| IBIS file stm32mp211_213_215_vfbga225.ibs
[IBIS ver] 5.1
[File name] stm32mp211_213_215_vfbga225.ibs
[File Rev] 0.4
[Date] 09-10-2025
[Source] Data Created at STMicroelectronics
[Notes]  File originated from ELDO simulations.
[Disclaimer]  This information is for modeling purpose only and is
   not guaranted. The information is subject to change without
   notice.
[Copyright] Copyright 2025 STMicroelectronics Inc.
|   Component stm32mp211_213_215_vfbga225
[Component] stm32mp211_213_215_vfbga225
[Manufacturer] STMicroelectronics
[Package]
| variable   typ   min   max
R_pkg  0  NA  NA
L_pkg  0  NA  NA
C_pkg  0  NA  NA
[Pin]   signal_name   model_name
A1  VSS  gnd
A2  PG5  io8_tt
A3  PG11  io8_tt
A4  PD3  io8_tt
A5  PD4  io8_tt
A6  PD15  io8_tt_i3c
A7  PE5  io8_tt
A8  PE3  io8_tt
A9  PE8  io8_tt
A10  PE13  io8_tt
A11  PE12  io8_tt
A12  PB14  io8_tt
A13  PD12  io8_tt
A14  PD13  io8_tt
A15  VSS  gnd
B1  PG7  io8_tt
B2  PI1  io8_tt_i3c
B3  PF15  io8_tt
B4  PD10  io8_tt_i3c
B5  PB11  io8_tt
B6  PD8  io8_tt
B7  PE1  io8_tt
B8  PE4  io8_tt
B9  PE15  io8_tt
B10  PE7  io8_tt
B11  PE9  io8_tt
B12  PB13  io8_tt
B13  PB12  io8_tt
B14  DDR_A20  mal4drv20_PAD
B15  DDR_DQ11  mal4drv27_PAD
C1  PF12  io8_tt
C2  PI4  io8_tt
C3  PF13  io8_tt
C4  PD2  io8_tt
C5  PD11  io8_tt_i3c
C6  PD1  io8_tt
C7  PD9  io8_tt
C8  PE0  io8_tt
C9  PE2  io8_tt
C10  PE11  io8_tt
C11  PD14  io8_tt
C12  DDR_RESETN  nc
C13  DDR_A9  mal4drv20_PAD
C14  DDR_A21  mal4drv20_PAD
C15  DDR_DQ9  mal4drv27_PAD
D1  OSC_OUT  isudq_v18
D2  OSC_IN  isudq_v18
D3  PI0  io8_tt
D4  PG12  io8_tt
D5  PD0  io8_tt
D6  PD7  io8_tt
D7  PD5  io8_tt
D8  PD6  io8_tt
D9  VDDA18PLL1  nc
D10  PE6  io8_tt
D11  DDR_A3  mal4drv20_PAD
D12  DDR_DQ10  mal4drv27_PAD
D13  DDR_A11  mal4drv20_PAD
D14  DDR_A22  mal4drv20_PAD
D15  DDR_DQS1N  mal4drv27_PAD
E1  OSC32_IN  isudq_v18
E2  OSC32_OUT  isudq_v18
E3  BOOT0  isudq_tt
E4  PC13  io8_tt
E5  VDDA18PLL2  nc
E6  VDDIO3  power
E7  VDDIO3  power
E8  VDDIO2  power
E9  VDDIO1  power
E10  VDDA18DDR  nc
E11  DDR_A0  mal4drv20_PAD
E12  DDR_DQ8  mal4drv27_PAD
E13  DDR_A10  mal4drv20_PAD
E14  DDR_A23  mal4drv20_PAD
E15  DDR_DQS1P  mal4drv27_PAD
F1  BOOT1  isudq_tt
F2  NRSTC1MS  io8_tt
F3  PWR_ON  io8_tt
F4  VDDA18AON  power
F5  VSSAON  nc
F6  VSS  gnd
F7  VDDCPU  nc
F8  VSS  gnd
F9  VDDCPU  nc
F10  VSS  gnd
F11  DDR_A5  mal4drv20_PAD
F12  DDR_A1  mal4drv20_PAD
F13  DDR_A8  mal4drv20_PAD
F14  DDR_A25  mal4drv20_PAD
F15  DDR_DQM1  mal4drv27_PAD
G1  JTDO_TRACESWO  io8_tt
G2  BOOT3  isudq_tt
G3  BOOT2  isudq_tt
G4  PDR_ON  nc
G5  V08CAP  nc
G6  VDDCORE  nc
G7  VSS  gnd
G8  VDDCPU  nc
G9  VSS  gnd
G10  VDDQDDR  power
G11  DDR_A4  mal4drv20_PAD
G12  DDR_DQ15  mal4drv27_PAD
G13  DDR_A14  mal4drv20_PAD
G14  DDR_A26  mal4drv20_PAD
G15  DDR_DQ12  mal4drv27_PAD
H1  JTCK_SWCLK  io8_tt
H2  NRST  nc
H3  PWR_LP  io8_tt
H4  PWR_CPUON  io8_tt
H5  VBAT  power
H6  VSS  gnd
H7  VDDCORE  nc
H8  VSS  gnd
H9  VDDQDDR  power
H10  VSS  gnd
H11  DDR_VREF  nc
H12  DDR_DQ5  mal4drv27_PAD
H13  DDR_DQ14  mal4drv27_PAD
H14  DDR_DQ13  mal4drv27_PAD
H15  DDR_DQ4  mal4drv27_PAD
J1  JTMS_SWDIO  io8_tt
J2  NJTRST  io8_tt
J3  JTDI  io8_tt
J4  VDDA18ADC  power
J5  VSSA  nc
J6  VDD  power
J7  VSS  gnd
J8  VDDCORE  nc
J9  VSS  gnd
J10  VDDQDDR  power
J11  DDR_A6  mal4drv20_PAD
J12  VSS  gnd
J13  DDR_ZQ  nc
J14  DDR_A13  mal4drv20_PAD
J15  DDR_DQ6  mal4drv27_PAD
K1  VREFN  nc
K2  PG2  io8_tt_i3c
K3  PA0  io8_tt
K4  PG3  io8_tt
K5  VDD  power
K6  VSS  gnd
K7  VDD  power
K8  VSS  gnd
K9  VDDCORE  nc
K10  VSS  gnd
K11  DDR_A18  mal4drv20_PAD
K12  DDR_DQ7  mal4drv27_PAD
K13  DDR_A27  mal4drv20_PAD
K14  DDR_A2  mal4drv20_PAD
K15  DDR_DQS0P  mal4drv27_PAD
L1  VREFP  nc
L2  PF11  io8_tt
L3  PG4  io8_tt
L4  PC8  io8_tt
L5  PF3  io8_tt
L6  PC0  io8_tt
L7  PH13  io8_tt
L8  PH11  io8_tt
L9  PA9  io8_tt
L10  VDDQDDR  power
L11  DDR_A31  mal4drv20_PAD
L12  DDR_A7  mal4drv20_PAD
L13  DDR_A28  mal4drv20_PAD
L14  DDR_A15  mal4drv20_PAD
L15  DDR_DQS0N  mal4drv27_PAD
M1  PB15  io8_tt
M2  PG1  io8_tt_i3c
M3  PC3  io8_tt
M4  PC9  io8_tt
M5  PC4  io8_tt
M6  PA15  io8_tt_i3c
M7  PA14  io8_tt
M8  PF0  io8_tt_i3c
M9  PA5  io8_tt
M10  PA2  io8_tt_i3c
M11  DDR_A12  mal4drv20_PAD
M12  DDR_DQM0  mal4drv27_PAD
M13  DDR_A29  mal4drv20_PAD
M14  DDR_A16  mal4drv20_PAD
M15  DDR_DQ0  mal4drv27_PAD
N1  PF4  io8_tt
N2  PF6  io8_tt
N3  PA10  io8_tt
N4  PF5  io8_tt
N5  PF8  io8_tt
N6  PC2  io8_tt
N7  PH9  io8_tt
N8  PA13  io8_tt
N9  PA8  io8_tt_i3c
N10  PA1  io8_tt_i3c
N11  DDR_DQ3  mal4drv27_PAD
N12  DDR_DQ2  mal4drv27_PAD
N13  DDR_A30  mal4drv20_PAD
N14  DDR_A17  mal4drv20_PAD
N15  DDR_DQ1  mal4drv27_PAD
P1  PF9  io8_tt
P2  PH4  io8_tt
P3  PF10  io8_tt
P4  PG0  io8_tt_i3c
P5  PF7  io8_tt
P6  PC5  io8_tt_i3c
P7  PC6  io8_tt_i3c
P8  PF2  io8_tt_i3c
P9  PH12  io8_tt
P10  PA7  io8_tt
P11  PH5  io8_tt
P12  PA3  io8_tt_i3c
P13  VSS  gnd
P14  OTG_HSDP  USB2_HS_IBIS
P15  VDD33USB  power
R1  VSS  gnd
R2  PC12  io8_tt_i3c
R3  PC11  io8_tt
R4  PA11  io8_tt
R5  PC7  io8_tt
R6  PC10  io8_tt
R7  PC1  io8_tt_i3c
R8  PF1  io8_tt
R9  PH10  io8_tt
R10  PA6  io8_tt
R11  PA4  io8_tt
R12  VDDA18USB  nc
R13  OTG_TXRTUNE  nc
R14  OTG_HSDM  USB2_HS_IBIS
R15  VSS  gnd
[Package Model]   503-fcvfbga-8x8-225-240814
[Pin Mapping]   pulldown_ref   pullup_ref   | Comment
A1  gnd  nc
A2  gnd  vdd
A3  gnd  vdd
A4  gnd  vddio3
A5  gnd  vddio3
A6  gnd  vdd
A7  gnd  vddio1
A8  gnd  vddio1
A9  gnd  vddio1
A10  gnd  vddio2
A11  gnd  vddio2
A12  gnd  vdd
A13  gnd  vdd
A14  gnd  vdd
A15  gnd  nc
B1  gnd  vdd
B2  gnd  vdd
B3  gnd  vdd
B4  gnd  vddio3
B5  gnd  vdd
B6  gnd  vddio3
B7  gnd  vddio1
B8  gnd  vddio1
B9  gnd  vddio2
B10  gnd  vddio1
B11  gnd  vddio1
B12  gnd  vdd
B13  gnd  vdd
B14  gnd  vddqddr
B15  gnd  vddqddr
C1  gnd  vdd
C2  gnd  vdd
C3  gnd  vdd
C4  gnd  vddio3
C5  gnd  vddio3
C6  gnd  vddio3
C7  gnd  vddio3
C8  gnd  vddio1
C9  gnd  vddio1
C10  gnd  vddio2
C11  gnd  vdd
C12  nc  nc
C13  gnd  vddqddr
C14  gnd  vddqddr
C15  gnd  vddqddr
D1  gnd  vdda18aon
D2  gnd  vdda18aon
D3  gnd  vdd
D4  gnd  vdd
D5  gnd  vddio3
D6  gnd  vddio3
D7  gnd  vddio3
D8  gnd  vddio3
D9  nc  nc
D10  gnd  vddio1
D11  gnd  vddqddr
D12  gnd  vddqddr
D13  gnd  vddqddr
D14  gnd  vddqddr
D15  gnd  vddqddr
E1  gnd  vdd  | Depending on IO usage
| E1  gnd  vsw  | Depending on IO usage
E2  gnd  vdd  | Depending on IO usage
| E2  gnd  vsw  | Depending on IO usage
E3  gnd  vdd
E4  gnd  vdd  | Depending on IO usage
| E4  gnd  vsw  | Depending on IO usage
E5  nc  nc
E6  nc  vddio3
E7  nc  vddio3
E8  nc  vddio2
E9  nc  vddio1
E10  nc  nc
E11  gnd  vddqddr
E12  gnd  vddqddr
E13  gnd  vddqddr
E14  gnd  vddqddr
E15  gnd  vddqddr
F1  gnd  vdd
F2  gnd  vdd
F3  gnd  vdd
F4  nc  vdda18aon
F5  nc  nc
F6  gnd  nc
F7  nc  nc
F8  gnd  nc
F9  nc  nc
F10  gnd  nc
F11  gnd  vddqddr
F12  gnd  vddqddr
F13  gnd  vddqddr
F14  gnd  vddqddr
F15  gnd  vddqddr
G1  gnd  vdd
G2  gnd  vdd
G3  gnd  vdd
G4  nc  nc
G5  nc  nc
G6  nc  nc
G7  gnd  nc
G8  nc  nc
G9  gnd  nc
G10  nc  vddqddr
G11  gnd  vddqddr
G12  gnd  vddqddr
G13  gnd  vddqddr
G14  gnd  vddqddr
G15  gnd  vddqddr
H1  gnd  vdd
H2  nc  nc
H3  gnd  vdd
H4  gnd  vdd
H5  nc  vsw
H6  gnd  nc
H7  nc  nc
H8  gnd  nc
H9  nc  vddqddr
H10  gnd  nc
H11  nc  nc
H12  gnd  vddqddr
H13  gnd  vddqddr
H14  gnd  vddqddr
H15  gnd  vddqddr
J1  gnd  vdd
J2  gnd  vdd
J3  gnd  vdd
J4  nc  vdda18adc
J5  nc  nc
J6  nc  vdd
J7  gnd  nc
J8  nc  nc
J9  gnd  nc
J10  nc  vddqddr
J11  gnd  vddqddr
J12  gnd  nc
J13  nc  nc
J14  gnd  vddqddr
J15  gnd  vddqddr
K1  nc  nc
K2  gnd  vdd
K3  gnd  vdd
K4  gnd  vdd
K5  nc  vdd
K6  gnd  nc
K7  nc  vdd
K8  gnd  nc
K9  nc  nc
K10  gnd  nc
K11  gnd  vddqddr
K12  gnd  vddqddr
K13  gnd  vddqddr
K14  gnd  vddqddr
K15  gnd  vddqddr
L1  nc  nc
L2  gnd  vdd
L3  gnd  vdd
L4  gnd  vdd
L5  gnd  vdd
L6  gnd  vdd
L7  gnd  vdd
L8  gnd  vdd
L9  gnd  vdd
L10  nc  vddqddr
L11  gnd  vddqddr
L12  gnd  vddqddr
L13  gnd  vddqddr
L14  gnd  vddqddr
L15  gnd  vddqddr
M1  gnd  vdd
M2  gnd  vdd
M3  gnd  vdd
M4  gnd  vdd
M5  gnd  vdd
M6  gnd  vdd
M7  gnd  vdd
M8  gnd  vdd
M9  gnd  vdd
M10  gnd  vdd
M11  gnd  vddqddr
M12  gnd  vddqddr
M13  gnd  vddqddr
M14  gnd  vddqddr
M15  gnd  vddqddr
N1  gnd  vdd
N2  gnd  vdd
N3  gnd  vdd
N4  gnd  vdd
N5  gnd  vdd
N6  gnd  vdd
N7  gnd  vdd
N8  gnd  vdd
N9  gnd  vdd
N10  gnd  vdd
N11  gnd  vddqddr
N12  gnd  vddqddr
N13  gnd  vddqddr
N14  gnd  vddqddr
N15  gnd  vddqddr
P1  gnd  vdd
P2  gnd  vdd
P3  gnd  vdd
P4  gnd  vdd
P5  gnd  vdd
P6  gnd  vdd
P7  gnd  vdd
P8  gnd  vdd
P9  gnd  vdd
P10  gnd  vdd
P11  gnd  vdd
P12  gnd  vdd
P13  gnd  nc
P14  gnd  vdd33usb
P15  nc  vdd33usb
R1  gnd  nc
R2  gnd  vdd
R3  gnd  vdd
R4  gnd  vdd
R5  gnd  vdd
R6  gnd  vdd
R7  gnd  vdd
R8  gnd  vdd
R9  gnd  vdd
R10  gnd  vdd
R11  gnd  vdd
R12  nc  nc
R13  nc  nc
R14  gnd  vdd33usb
R15  gnd  nc
[Diff Pin]  inv_pin  vdiff  tdelay_typ  tdelay_min  tdelay_max
K15  L15  NA  NA  NA  NA
E15  D15  NA  NA  NA  NA
G11  F11  NA  NA  NA  NA
P14  R14  NA  NA  NA  NA   |USBH_HS_DP _DM
[Model Selector] USB2_HS_IBIS
USB2_HSRX   USB2 HSRX model
USB2_HSTX_00_0_01_0011_11   TuningBits_AMP_PULSE_RISE_REF_XV=00_0_01_0011_11
USB2_HSTX_00_0_10_0101_11   TuningBits_AMP_PULSE_RISE_REF_XV=00_0_10_0101_11
USB2_HSTX_00_0_11_0111_11   TuningBits_AMP_PULSE_RISE_REF_XV=00_0_11_0111_11
USB2_HSTX_00_1_01_0011_11   TuningBits_AMP_PULSE_RISE_REF_XV=00_1_01_0011_11
USB2_HSTX_00_1_10_0101_11   TuningBits_AMP_PULSE_RISE_REF_XV=00_1_10_0101_11
USB2_HSTX_00_1_11_0111_11   TuningBits_AMP_PULSE_RISE_REF_XV=00_1_11_0111_11
USB2_HSTX_01_0_01_0011_11   TuningBits_AMP_PULSE_RISE_REF_XV=01_0_01_0011_11
USB2_HSTX_01_0_10_0101_11   TuningBits_AMP_PULSE_RISE_REF_XV=01_0_10_0101_11
USB2_HSTX_01_0_11_0111_11   TuningBits_AMP_PULSE_RISE_REF_XV=01_0_11_0111_11
USB2_HSTX_01_1_01_0011_11   TuningBits_AMP_PULSE_RISE_REF_XV=01_1_01_0011_11
USB2_HSTX_01_1_10_0101_11   TuningBits_AMP_PULSE_RISE_REF_XV=01_1_10_0101_11
USB2_HSTX_01_1_11_0111_11   TuningBits_AMP_PULSE_RISE_REF_XV=01_1_11_0111_11
USB2_HSTX_10_0_01_0011_11   TuningBits_AMP_PULSE_RISE_REF_XV=10_0_01_0011_11
USB2_HSTX_10_0_10_0101_11   TuningBits_AMP_PULSE_RISE_REF_XV=10_0_10_0101_11
USB2_HSTX_10_0_11_0111_11   TuningBits_AMP_PULSE_RISE_REF_XV=10_0_11_0111_11
USB2_HSTX_10_1_01_0011_11   TuningBits_AMP_PULSE_RISE_REF_XV=10_1_01_0011_11
USB2_HSTX_10_1_10_0101_11   TuningBits_AMP_PULSE_RISE_REF_XV=10_1_10_0101_11
USB2_HSTX_10_1_11_0111_11   TuningBits_AMP_PULSE_RISE_REF_XV=10_1_11_0111_11
[Model Selector] io8_tt
io8_tt_ls_3v3 "GPIO - 3V tolerant - low speed - 3.3V range"
io8_tt_ms_3v3 "GPIO - 3V tolerant - med speed - 3.3V range"
io8_tt_fs_3v3 "GPIO - 3V tolerant - fast speed - 3.3V range"
io8_tt_hs_3v3 "GPIO - 3V tolerant - high speed - 3.3V range"
io8_tt_hslv_ls_1v8 "GPIO low voltage optimization - 3V tolerant - low speed - 1.8V range"
io8_tt_hslv_ms_1v8 "GPIO low voltage optimization - 3V tolerant - med speed - 1.8V range"
io8_tt_hslv_fs_1v8 "GPIO low voltage optimization - 3V tolerant - fast speed - 1.8V range"
io8_tt_hslv_hs_1v8 "GPIO low voltage optimization - 3V tolerant - high speed - 1.8V range"
[Model Selector] io8_tt_i3c
io8_tt_ls_3v3 "GPIO - 3V tolerant - low speed - 3.3V range"
io8_tt_ms_3v3 "GPIO - 3V tolerant - med speed - 3.3V range"
io8_tt_fs_3v3 "GPIO - 3V tolerant - fast speed - 3.3V range"
io8_tt_hs_3v3 "GPIO - 3V tolerant - high speed - 3.3V range"
io8_tt_hslv_ls_1v8 "GPIO low voltage optimization - 3V tolerant - low speed - 1.8V range"
io8_tt_hslv_ms_1v8 "GPIO low voltage optimization - 3V tolerant - med speed - 1.8V range"
io8_tt_hslv_fs_1v8 "GPIO low voltage optimization - 3V tolerant - fast speed - 1.8V range"
io8_tt_hslv_hs_1v8 "GPIO low voltage optimization - 3V tolerant - high speed - 1.8V range"
io8_tt_i3c_ls_3v3 "GPIO with I3C open-drain - 3V tolerant - low speed - 3.3V range"
io8_tt_i3c_ms_3v3 "GPIO with I3C open-drain - 3V tolerant - med speed - 3.3V range"
io8_tt_i3c_fs_3v3 "GPIO with I3C open-drain - 3V tolerant - fast speed - 3.3V range"
io8_tt_i3c_hs_3v3 "GPIO with I3C open-drain - 3V tolerant - high speed - 3.3V range"
io8_tt_hslv_i3c_ls_1v8 "GPIO low voltage optimization with I3C open-drain - 3V tolerant - low speed - 1.8V range"
io8_tt_hslv_i3c_ms_1v8 "GPIO low voltage optimization with I3C open-drain - 3V tolerant - med speed - 1.8V range"
io8_tt_hslv_i3c_fs_1v8 "GPIO low voltage optimization with I3C open-drain - 3V tolerant - fast speed - 1.8V range"
io8_tt_hslv_i3c_hs_1v8 "GPIO low voltage optimization with I3C open-drain - 3V tolerant - high speed - 1.8V range"
io8_tt_i3c_fmp_3v3 "GPIO with I3C fm+ open-drain - 3V tolerant - 3.3V range"
[Model Selector] isudq_tt
isudq_tt_3v3 "Input Buffer - 3V tolerant - 3.3V range"
isudq_tt_1v8 "Input Buffer - 3V tolerant - 1.8V range"
|[Model Selector] isudq_v18
|isudq_v18_1v8 "Input Buffer - 1.8V range "
[Model Selector]   mal4drv20_PAD
mal4drv20_d3l_40   DDR3L mal4drv20 cell  Z0=40-Ohm Driver
mal4drv20_d3l_60   DDR3L mal4drv20 cell  Z0=60-Ohm Driver
mal4drv20_d3l_120   DDR3L mal4drv20 cell  Z0=120-Ohm Driver
mal4drv20_d3_20   DDR3 mal4drv20 cell  Z0=20-Ohm Driver
mal4drv20_d3_24   DDR3 mal4drv20 cell  Z0=24-Ohm Driver
mal4drv20_d3_30   DDR3 mal4drv20 cell  Z0=30-Ohm Driver
mal4drv20_d3_40   DDR3 mal4drv20 cell  Z0=40-Ohm Driver
mal4drv20_d3_60   DDR3 mal4drv20 cell  Z0=60-Ohm Driver
mal4drv20_d4_20   DDR4 mal4drv20 cell  Z0=20-Ohm Driver
mal4drv20_d4_24   DDR4 mal4drv20 cell  Z0=24-Ohm Driver
mal4drv20_d4_30   DDR4 mal4drv20 cell  Z0=30-Ohm Driver
mal4drv20_d4_40   DDR4 mal4drv20 cell  Z0=40-Ohm Driver
mal4drv20_d4_60   DDR4 mal4drv20 cell  Z0=60-Ohm Driver
mal4drv20_dl4_20   LPDDR4 mal4drv20 cell  Z0=20-Ohm Driver
mal4drv20_dl4_24   LPDDR4 mal4drv20 cell  Z0=24-Ohm Driver
mal4drv20_dl4_30   LPDDR4 mal4drv20 cell  Z0=30-Ohm Driver
mal4drv20_dl4_40   LPDDR4 mal4drv20 cell  Z0=40-Ohm Driver
mal4drv20_dl4_60   LPDDR4 mal4drv20 cell  Z0=60-Ohm Driver
[Model Selector]   mal4drv27_PAD
mal4drv27_d3l_40   DDR3L mal4drv27 cell  Z0=40-Ohm Driver
mal4drv27_d3l_48   DDR3L mal4drv27 cell  Z0=48-Ohm Driver
mal4drv27_d3l_60   DDR3L mal4drv27 cell  Z0=60-Ohm Driver
mal4drv27_d3l_80   DDR3L mal4drv27 cell  Z0=80-Ohm Driver
mal4drv27_d3l_120   DDR3L mal4drv27 cell  Z0=120-Ohm Driver
mal4drv27_d3l_240   DDR3L mal4drv27 cell  Z0=240-Ohm Driver
mal4drv27_d3l_odt120   DDR3L mal4drv27 cell 120-Ohm ODT Receiver
mal4drv27_d3l_odt60   DDR3L mal4drv27 cell 60-Ohm ODT Receiver
mal4drv27_d3l_odtoff   DDR3L mal4drv27 cell ODT OFF Receiver
mal4drv27_d3_28   DDR3 mal4drv27 cell  Z0=28-Ohm Driver
mal4drv27_d3_34   DDR3 mal4drv27 cell  Z0=34-Ohm Driver
mal4drv27_d3_40   DDR3 mal4drv27 cell  Z0=40-Ohm Driver
mal4drv27_d3_53   DDR3 mal4drv27 cell  Z0=53-Ohm Driver
mal4drv27_d3_odt120   DDR3 mal4drv27 cell 120-Ohm ODT Receiver
mal4drv27_d3_odt60   DDR3 mal4drv27 cell 60-Ohm ODT Receiver
mal4drv27_d4_28   DDR4 mal4drv27 cell  Z0=28-Ohm Driver
mal4drv27_d4_34   DDR4 mal4drv27 cell  Z0=34-Ohm Driver
mal4drv27_d4_40   DDR4 mal4drv27 cell  Z0=40-Ohm Driver
mal4drv27_d4_53   DDR4 mal4drv27 cell  Z0=53-Ohm Driver
mal4drv27_d4_odt120   DDR4 mal4drv27 cell 120-Ohm ODT Receiver
mal4drv27_d4_odt240   DDR4 mal4drv27 cell 240-Ohm ODT Receiver
mal4drv27_d4_odt48   DDR4 mal4drv27 cell 48-Ohm ODT Receiver
mal4drv27_d4_odt60   DDR4 mal4drv27 cell 60-Ohm ODT Receiver
mal4drv27_d4_odt80   DDR4 mal4drv27 cell 80-Ohm ODT Receiver
mal4drv27_dl4_28   LPDDR4 mal4drv27 cell  Z0=28-Ohm Driver
mal4drv27_dl4_34   LPDDR4 mal4drv27 cell  Z0=34-Ohm Driver
mal4drv27_dl4_40   LPDDR4 mal4drv27 cell  Z0=40-Ohm Driver
mal4drv27_dl4_53   LPDDR4 mal4drv27 cell  Z0=53-Ohm Driver
mal4drv27_dl4_odt48   LPDDR4 mal4drv27 cell 48-Ohm ODT Receiver
mal4drv27_dl4_odt60   LPDDR4 mal4drv27 cell 60-Ohm ODT Receiver
[Define Package Model]  503-fcvfbga-8x8-225-240814
[Manufacturer]  unknown
[OEM]  unknown
[Description]  unknown
[Number Of Pins]  196
[Pin Numbers]
| Pin Name Terminal   Net Name   Starting Node   Ending Node
E3 | BOOT0
F1 | BOOT1
G3 | BOOT2
G2 | BOOT3
E11 | DDR_A0
F12 | DDR_A1
K14 | DDR_A2
D11 | DDR_A3
G11 | DDR_A4
F11 | DDR_A5
J11 | DDR_A6
L12 | DDR_A7
F13 | DDR_A8
C13 | DDR_A9
E13 | DDR_A10
D13 | DDR_A11
M11 | DDR_A12
J14 | DDR_A13
G13 | DDR_A14
L14 | DDR_A15
M14 | DDR_A16
N14 | DDR_A17
K11 | DDR_A18
B14 | DDR_A20
C14 | DDR_A21
D14 | DDR_A22
E14 | DDR_A23
F14 | DDR_A25
G14 | DDR_A26
K13 | DDR_A27
L13 | DDR_A28
M13 | DDR_A29
N13 | DDR_A30
L11 | DDR_A31
M15 | DDR_DQ0
N15 | DDR_DQ1
N12 | DDR_DQ2
N11 | DDR_DQ3
H15 | DDR_DQ4
H12 | DDR_DQ5
J15 | DDR_DQ6
K12 | DDR_DQ7
E12 | DDR_DQ8
C15 | DDR_DQ9
D12 | DDR_DQ10
B15 | DDR_DQ11
G15 | DDR_DQ12
H14 | DDR_DQ13
H13 | DDR_DQ14
G12 | DDR_DQ15
M12 | DDR_DQM0
F15 | DDR_DQM1
L15 | DDR_DQS0N
K15 | DDR_DQS0P
D15 | DDR_DQS1N
E15 | DDR_DQS1P
C12 | DDR_RESETN
H11 | DDR_VREF
J13 | DDR_ZQ
H1 | JTCK_SWCLK
J3 | JTDI
G1 | JTDO_TRACESWO
J1 | JTMS_SWDIO
J2 | NJTRST
H2 | NRST
F2 | NRSTC1MS
E1 | OSC32_IN
E2 | OSC32_OUT
D2 | OSC_IN
D1 | OSC_OUT
R14 | OTG_HSDM
P14 | OTG_HSDP
R13 | OTG_TXRTUNE
K3 | PA0
N10 | PA1
M10 | PA2
P12 | PA3
R11 | PA4
M9 | PA5
R10 | PA6
P10 | PA7
N9 | PA8
L9 | PA9
N3 | PA10
R4 | PA11
N8 | PA13
M7 | PA14
M6 | PA15
B5 | PB11
B13 | PB12
B12 | PB13
A12 | PB14
M1 | PB15
L6 | PC0
R7 | PC1
N6 | PC2
M3 | PC3
M5 | PC4
P6 | PC5
P7 | PC6
R5 | PC7
L4 | PC8
M4 | PC9
R6 | PC10
R3 | PC11
R2 | PC12
E4 | PC13
D5 | PD0
C6 | PD1
C4 | PD2
A4 | PD3
A5 | PD4
D7 | PD5
D8 | PD6
D6 | PD7
B6 | PD8
C7 | PD9
B4 | PD10
C5 | PD11
A13 | PD12
A14 | PD13
C11 | PD14
A6 | PD15
G4 | PDR_ON
C8 | PE0
B7 | PE1
C9 | PE2
A8 | PE3
B8 | PE4
A7 | PE5
D10 | PE6
B10 | PE7
A9 | PE8
B11 | PE9
C10 | PE11
A11 | PE12
A10 | PE13
B9 | PE15
M8 | PF0
R8 | PF1
P8 | PF2
L5 | PF3
N1 | PF4
N4 | PF5
N2 | PF6
P5 | PF7
N5 | PF8
P1 | PF9
P3 | PF10
L2 | PF11
C1 | PF12
C3 | PF13
B3 | PF15
P4 | PG0
M2 | PG1
K2 | PG2
K4 | PG3
L3 | PG4
A2 | PG5
B1 | PG7
A3 | PG11
D4 | PG12
P2 | PH4
P11 | PH5
N7 | PH9
R9 | PH10
L8 | PH11
P9 | PH12
L7 | PH13
D3 | PI0
B2 | PI1
C2 | PI4
H4 | PWR_CPUON
H3 | PWR_LP
F3 | PWR_ON
G5 | V08CAP
H5 | VBAT
P15 | VDD33USB
J6 | VDD
J4 | VDDA18ADC
F4 | VDDA18AON
E10 | VDDA18DDR
D9 | VDDA18PLL1
E5 | VDDA18PLL2
R12 | VDDA18USB
G6 | VDDCORE
F7 | VDDCPU
E9 | VDDIO1
E8 | VDDIO2
E6 | VDDIO3
G10 | VDDQDDR
K1 | VREFN
L1 | VREFP
A1 | VSS
J5 | VSSA
F5 | VSSAON
|[Merged Pins]  J6
|K5  |  VDD
|K7  |  VDD
|[Merged Pins]  G6
|H7  |  VDDCORE
|J8  |  VDDCORE
|K9  |  VDDCORE
|[Merged Pins]  F7
|F9  |  VDDCPU
|G8  |  VDDCPU
|[Merged Pins]  E6
|E7  |  VDDIO3
|[Merged Pins]  G10
|H9  |  VDDQDDR
|J10  |  VDDQDDR
|L10  |  VDDQDDR
|[Merged Pins]  A1
|A15  |  VSS
|F6  |  VSS
|F8  |  VSS
|F10  |  VSS
|G7  |  VSS
|G9  |  VSS
|H6  |  VSS
|H8  |  VSS
|H10  |  VSS
|J7  |  VSS
|J9  |  VSS
|J12  |  VSS
|K6  |  VSS
|K8  |  VSS
|K10  |  VSS
|P13  |  VSS
|R1  |  VSS
|R15  |  VSS
[Model Data]
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[End Model Data]
[End Package Model]
|End [Component]
| Models and submodels in the file (87): USB2_HSRX (Input), USB2_HSTX_00_0_01_0011_11 (Output), USB2_HSTX_00_0_10_0101_11 (Output), USB2_HSTX_00_0_11_0111_11 (Output), USB2_HSTX_00_1_01_0011_11 (Output), USB2_HSTX_00_1_10_0101_11 (Output), USB2_HSTX_00_1_11_0111_11 (Output), USB2_HSTX_01_0_01_0011_11 (Output), USB2_HSTX_01_0_10_0101_11 (Output), USB2_HSTX_01_0_11_0111_11 (Output), USB2_HSTX_01_1_01_0011_11 (Output), USB2_HSTX_01_1_10_0101_11 (Output), USB2_HSTX_01_1_11_0111_11 (Output), USB2_HSTX_10_0_01_0011_11 (Output), USB2_HSTX_10_0_10_0101_11 (Output), USB2_HSTX_10_0_11_0111_11 (Output), USB2_HSTX_10_1_01_0011_11 (Output), USB2_HSTX_10_1_10_0101_11 (Output), USB2_HSTX_10_1_11_0111_11 (Output), mal4drv20_d3_20 (I/O), mal4drv20_d3_24 (I/O), mal4drv20_d3_30 (I/O), mal4drv20_d3_40 (I/O), mal4drv20_d3_60 (I/O), mal4drv20_d4_20 (I/O), mal4drv20_d4_24 (I/O), mal4drv20_d4_30 (I/O), mal4drv20_d4_40 (I/O), mal4drv20_d4_60 (I/O), mal4drv20_dl4_20 (I/O), mal4drv20_dl4_24 (I/O), mal4drv20_dl4_30 (I/O), mal4drv20_dl4_40 (I/O), mal4drv20_dl4_60 (I/O), mal4drv27_d3_28 (I/O), mal4drv27_d3_34 (I/O), mal4drv27_d3_40 (I/O), mal4drv27_d3_53 (I/O), mal4drv27_d3_odt120 (Input), mal4drv27_d3_odt60 (Input), mal4drv27_dl4_28 (I/O), mal4drv27_dl4_34 (I/O), mal4drv27_dl4_40 (I/O), mal4drv27_dl4_53 (I/O), mal4drv27_dl4_odt48 (Input), mal4drv27_dl4_odt60 (Input), mal4drv27_d4_28 (I/O), mal4drv27_d4_34 (I/O), mal4drv27_d4_40 (I/O), mal4drv27_d4_53 (I/O), mal4drv27_d4_odt120 (Input), mal4drv27_d4_odt240 (Input), mal4drv27_d4_odt48 (Input), mal4drv27_d4_odt60 (Input), mal4drv27_d4_odt80 (Input), mal4drv20_d3l_120 (I/O), mal4drv20_d3l_40 (I/O), mal4drv20_d3l_60 (I/O), mal4drv27_d3l_120 (I/O), mal4drv27_d3l_240 (I/O), mal4drv27_d3l_40 (I/O), mal4drv27_d3l_48 (I/O), mal4drv27_d3l_60 (I/O), mal4drv27_d3l_80 (I/O), mal4drv27_d3l_odt120 (Input), mal4drv27_d3l_odt60 (Input), mal4drv27_d3l_odtoff (Input), io8_tt_fs_3v3 (I/O), io8_tt_hs_3v3 (I/O), io8_tt_hslv_fs_1v8 (I/O), io8_tt_hslv_hs_1v8 (I/O), io8_tt_hslv_i3c_fs_1v8 (I/O_open_drain), io8_tt_hslv_i3c_hs_1v8 (I/O_open_drain), io8_tt_hslv_i3c_ls_1v8 (I/O_open_drain), io8_tt_hslv_i3c_ms_1v8 (I/O_open_drain), io8_tt_hslv_ls_1v8 (I/O), io8_tt_hslv_ms_1v8 (I/O), io8_tt_i3c_fmp_3v3 (I/O_open_drain), io8_tt_i3c_fs_3v3 (I/O_open_drain), io8_tt_i3c_hs_3v3 (I/O_open_drain)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
